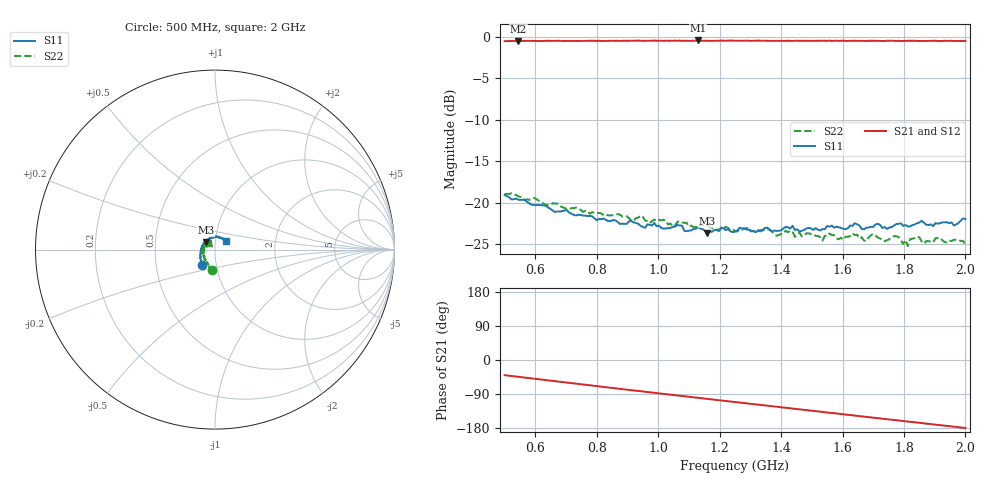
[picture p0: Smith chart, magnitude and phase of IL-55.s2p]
!Agilent Technologies,E8361C,US49010292,A.09.42.06
!Agilent E8361C: A.09.42.06
!Date: Monday, January 13, 2025 00:07:31
!Correction: S11(Full 2 Port(1,2))
!S21(Full 2 Port(1,2))
!S12(Full 2 Port(1,2))
!S22(Full 2 Port(1,2))
!S2P File: Measurements: S11, S21, S12, S22:
# Hz S  dB  R 50
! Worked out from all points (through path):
!   201 points, 500 MHz to 2 GHz, reference 50 ohm
!   highest |S21| = -0.43 dB at 1.13 GHz (marker M1); lowest = -0.5 dB at 545 MHz (marker M2)
!   group delay of S21, straight-line fit = 257 ps
!   lowest |S11| = -23.7 dB at 1.16 GHz (marker M3), VSWR 1.14, Z = 45.1 + j3.77 ohm
!   |S11| at or under -10 dB: start of sweep to end of sweep
!   |S22| runs from -25.2 to -18.9 dB; largest |S21 - S12| = 0.006
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5e8  -19.07 -131.0  -0.51 -40.1  -0.52 -40.2  -18.94 -97.7
5.45e8  -19.64 -135.0  -0.51 -44.6  -0.50 -44.5  -19.24 -103.7
7.55e8  -21.55 -164.4  -0.46 -64.9  -0.48 -64.8  -21.09 -117.2
1.0025e9  -22.75 161.4  -0.47 -88.1  -0.47 -88.1  -22.07 -134.6
1.13e9  -22.96 146.4  -0.43 -99.9  -0.48 -99.8  -23.11 -146.3
1.16e9  -23.69 140.4  -0.47 -102.6  -0.47 -102.6  -22.77 -150.2
1.25e9  -23.48 129.2  -0.47 -111.1  -0.49 -110.9  -23.39 -159.2
1.505e9  -23.29 96.8  -0.48 -134.3  -0.46 -134.3  -23.78 178.3
1.535e9  -23.18 94.3  -0.46 -137.0  -0.47 -137.1  -24.56 178.2
1.5575e9  -22.90 91.8  -0.45 -139.1  -0.48 -139.2  -23.72 175.6
1.6025e9  -23.14 84.8  -0.46 -143.2  -0.47 -143.3  -24.48 172.9
1.6325e9  -22.79 84.1  -0.46 -146.1  -0.50 -146.0  -23.70 168.4
1.67e9  -23.21 76.6  -0.47 -149.3  -0.47 -149.3  -24.57 165.8
1.7e9  -22.90 74.2  -0.47 -152.3  -0.48 -152.1  -23.75 162.6
1.7525e9  -22.99 67.0  -0.47 -156.9  -0.49 -156.9  -24.38 160.0
1.775e9  -22.57 65.2  -0.49 -158.9  -0.50 -159.2  -24.04 154.7
1.8125e9  -22.87 59.0  -0.46 -162.4  -0.47 -162.4  -25.24 153.3
1.82e9  -22.85 61.3  -0.46 -163.2  -0.50 -163.1  -24.39 152.4
1.8425e9  -22.47 59.3  -0.48 -165.1  -0.48 -165.0  -24.09 147.7
1.865e9  -22.40 53.3  -0.49 -167.2  -0.50 -167.2  -24.94 148.1
1.9175e9  -22.47 50.3  -0.50 -171.9  -0.47 -171.9  -24.23 139.6
2e9  -21.97 39.5  -0.48 -179.3  -0.49 -179.2  -25.07 136.1
